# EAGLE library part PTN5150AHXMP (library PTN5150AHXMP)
USB Controller USB Interface 12-X2QFN (1.6x1.6), 2.7V ~ 5.5V , 100 uA , -40C ~ 85C Source: Datasheet
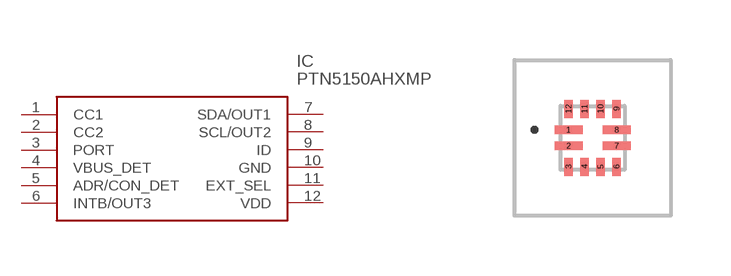
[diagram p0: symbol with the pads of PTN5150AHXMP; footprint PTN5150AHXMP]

Designator prefix IC

## PTN5150AHXMP (Description: USB Controller USB Interface 12-X2QFN (1.6x1.6), 2.7V ~ 5.5V , 100 uA , -40C ~ 85C; Height: 0.4mm; Manufacturer_Name: NXP; Manufacturer_Part_Number: PTN5150AHXMP; Mouser_Part_Number: 771-PTN5150AHXMP; Mouser_Price-Stock: https://www.mouser.co.uk/ProductDetail/NXP-Semiconductors/PTN5150AHXMP?qs=GIi83qBHgikdzCs4%252ByCwLg%3D%3D)  [PTN5150AHXMP]
1  CC1
2  CC2
3  PORT
4  VBUS_DET
5  ADR/CON_DET
6  INTB/OUT3
7  SDA/OUT1
8  SCL/OUT2
9  ID
10  GND
11  EXT_SEL
12  VDD

## Footprint PTN5150AHXMP (pad centres in mm)
SOT1355-1_2025
smd 0.7 x 0.22: 1 -0.6,0.2; 2 -0.6,-0.2; 7 0.6,-0.2; 8 0.6,0.2
smd 0.22 x 0.45: 3 -0.6,-0.725; 4 -0.2,-0.725; 5 0.2,-0.725; 6 0.6,-0.725; 9 0.6,0.725; 10 0.2,0.725; 11 -0.2,0.725; 12 -0.6,0.725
